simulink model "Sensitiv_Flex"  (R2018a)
settings: Solver=ode113  StartTime=0.0  StopTime=20  FixedStep=0.0001  RelTol=1e-5  EnableMultiTasking=on
InitFcn:
  | init
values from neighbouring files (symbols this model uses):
  d2r = pi/180    (= 0.0174532925199)    [init.m]    (also in LQR_Design.m)
  Kr = Kq; Kr(3)=-Kq(3)    [init.m]
  r2d = 1/d2r    (= 57.2957795131)    [init.m]    (also in LQR_Design.m)
  Wf = 18    [init.m]
undefined symbols (not defined in the file or in its folder): Aa, Av, Ba, Bv, Ca, Cv, Da, Dv, Kq, TVC

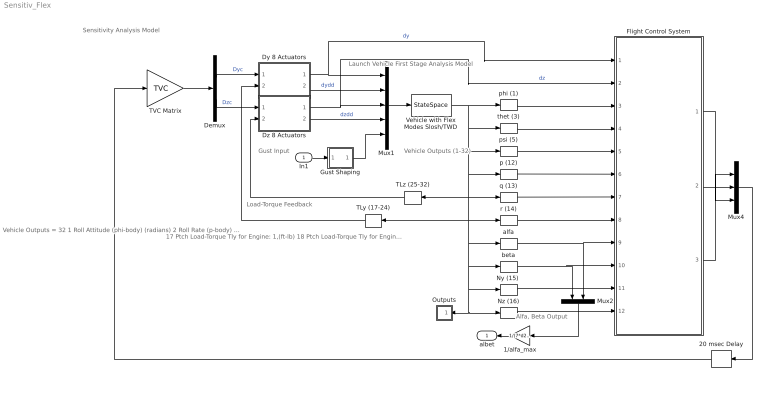
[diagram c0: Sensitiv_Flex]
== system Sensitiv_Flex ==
  note: Gust Input
  note: Launch Vehicle First Stage Analysis Model
  note: Load-Torque Feedback
  note: 17 Ptch Load-Torque Tly for Engine: 1,(ft-lb) 18 Ptch Load-Torque Tly for Engine: 2,(ft-lb) 19 Ptch Load-Torque Tly for Engine: 3,(ft-lb) 20 Ptch Load-Torque Tly for Engine: 4,(ft-lb) 21 Ptch Load-Torque Tly for Engine: 5,(ft-lb) 22 Ptch Load-Torque Tly for Engine: 6,(ft-lb) 23 Ptch Load-Torque Tly for Engine: 7,(ft-lb) 24 Ptch Load-Torque Tly for Engine: 8,(ft-lb) 25 Yaw Load-Torque Tlz for Engine: 1,(ft-lb) 26 Yaw Load-Torque Tlz for Engine: 2,(ft-lb) 27 Yaw Load-Torque Tlz for Engine: 3,(ft-lb) 28 Yaw Load-Torque Tlz for Engine: 4,(ft-lb) 29 Yaw Load-Torque Tlz for Engine: 5,(ft-lb) 30 Yaw Load-Torque Tlz for Engine: 6,(ft-lb) 31 Yaw Load-Torque Tlz for Engine: 7,(ft-lb) 32 Yaw Load-Torque Tlz for Engine: 8,(ft-lb)
  note: Vehicle Outputs = 32 1 Roll Attitude (phi-body) (radians) 2 Roll Rate (p-body) (rad/sec) 3 Pitch Attitude (thet-bdy) (radians) 4 Pitch Rate (q-body) (rad/sec) 5 Yaw Attitude (psi-body) (radians) 6 Yaw Rate (r-body) (rad/sec) 7 Angle of attack, alfa, (radians) 8 Angle of sideslip, beta, (radian) 9 Change in Altitude, delta-h, (feet) 10 Forward Acceleration (V-dot) (ft/sec) 11 Cross Range Velocity (Vcr) (ft/sec) 12 Rate-Gyro # 1, Roll Rate (Body) (rad/sec) 13 Rate-Gyro # 2, Pitch Rate (Body) (rad/sec) 14 Rate-Gyro # 3, Yaw Rate (Body) (rad/sec) 15 Accelerom # 1, (along Y), (ft/sec^2) Translat. Accelerat. 16 Accelerom # 2, (along Z), (ft/sec^2) Translat. Accelerat.
  note: Vehicle Outputs (1-32)
  note: Sensitivity Analysis Model
  note: Alfa, Beta Output
  In1 : Inport
  1/alfa_max : Gain  Gain=1/(7*d2r)
  20 msec Delay : TransportDelay  DelayTime="[1  1  1]*0.02"  InitialOutput="[0  0  0]"  PadeOrder=2
  Demux : Demux  Outputs=[8, 8]
  Dy 8 Actuators : Subsystem
  Dz 8 Actuators : Subsystem
  Flight Control System : Subsystem
  Gust Shaping : Subsystem
  Mux1 : Mux  Inputs=[8, 8, 8, 8, 1]
  Mux2 : Mux  Inputs=2
  Mux4 : Mux  Inputs=3
  "Ny (15) " : Selector  InputPortWidth=32  IndexOptions=Index vector (dialog)  Indices=[15]  OutputSizes=1
  Nz (16) : Selector  InputPortWidth=32  IndexOptions=Index vector (dialog)  Indices=[16]  OutputSizes=1
  Outputs : Subsystem
  TLy (17-24) : Selector  InputPortWidth=32  IndexOptions=Index vector (dialog)  Indices=[17:24]  OutputSizes=1
  TLz (25-32) : Selector  InputPortWidth=32  IndexOptions=Index vector (dialog)  Indices=[25:32]  OutputSizes=1
  TVC Matrix : Gain  Gain=TVC  Multiplication=Matrix(K*u)
  Vehicle with Flex Modes Slosh/TWD : StateSpace  A=Av  B=Bv  C=Cv  D=Dv  InitialCondition=0
  alfa : Selector  InputPortWidth=32  IndexOptions=Index vector (dialog)  Indices=[7]  OutputSizes=1
  beta : Selector  InputPortWidth=32  IndexOptions=Index vector (dialog)  Indices=[8]  OutputSizes=1
  p (12) : Selector  InputPortWidth=32  IndexOptions=Index vector (dialog)  Indices=[12]  OutputSizes=1
  phi (1) : Selector  InputPortWidth=32  IndexOptions=Index vector (dialog)  Indices=[1]  OutputSizes=1
  psi (5) : Selector  InputPortWidth=32  IndexOptions=Index vector (dialog)  Indices=[5]  OutputSizes=1
  q (13) : Selector  InputPortWidth=32  IndexOptions=Index vector (dialog)  Indices=[13]  OutputSizes=1
  r (14) : Selector  InputPortWidth=32  IndexOptions=Index vector (dialog)  Indices=[14]  OutputSizes=1
  thet (3) : Selector  InputPortWidth=32  IndexOptions=Index vector (dialog)  Indices=[3]  OutputSizes=1
  albet : Outport
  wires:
  Mux1/1 -> Vehicle with Flex Modes Slosh/TWD/1
  Dy 8 Actuators/2(dydd) -> Mux1/2  "dydd"
  Dz 8 Actuators/2(dzdd) -> Mux1/4  "dzdd"
  Demux/1 -> Dy 8 Actuators/1(dyc)  "Dyc"
  Dy 8 Actuators/1(dy) -> Flight Control System/1(dy), Mux1/1  "dy"
  Dz 8 Actuators/1(dz) -> Flight Control System/2(dz), Mux1/3  "dz"
  Demux/2 -> Dz 8 Actuators/1(dzc)  "Dzc"
  TLy (17-24)/1 -> Dy 8 Actuators/2(TLy)
  TLz (25-32)/1 -> Dz 8 Actuators/2(TLz)
  Vehicle with Flex Modes Slosh/TWD/1 -> TLz (25-32)/1, "Ny (15) "/1, Outputs/1(in), Nz (16)/1, beta/1, alfa/1, TLy (17-24)/1, r (14)/1, q (13)/1, p (12)/1, psi (5)/1, thet (3)/1, phi (1)/1
  r (14)/1 -> Flight Control System/8(r)
  q (13)/1 -> Flight Control System/7(q)
  p (12)/1 -> Flight Control System/6(p)
  Mux4/1 -> 20 msec Delay/1
  alfa/1 -> Flight Control System/9(alfa), Mux2/2
  beta/1 -> Flight Control System/10(beta), Mux2/1
  "Ny (15) "/1 -> Flight Control System/11(NY)
  Nz (16)/1 -> Flight Control System/12(NZ)
  Flight Control System/2(DQ_tvc) -> Mux4/2
  Flight Control System/1(DP_tvc) -> Mux4/1
  Flight Control System/3(DR_tvc) -> Mux4/3
  phi (1)/1 -> Flight Control System/3(phi)
  thet (3)/1 -> Flight Control System/4(thet)
  psi (5)/1 -> Flight Control System/5(psi)
  TVC Matrix/1 -> Demux/1
  In1/1 -> Gust Shaping/1(i)
  Mux2/1 -> 1/alfa_max/1
  20 msec Delay/1 -> TVC Matrix/1
  Gust Shaping/1(o) -> Mux1/5
  1/alfa_max/1 -> albet/1

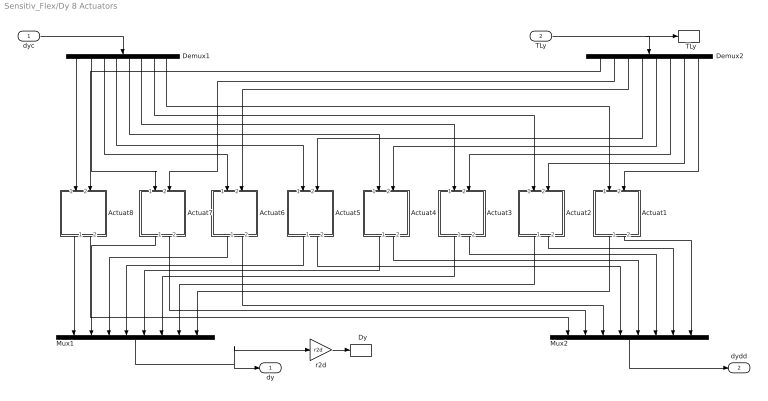
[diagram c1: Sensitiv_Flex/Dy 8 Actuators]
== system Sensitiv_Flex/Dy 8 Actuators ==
  dyc : Inport
  TLy : Inport  Port=2
  "  Dy" : ToWorkspace  VariableName=DY  SampleTime=-1
  "  TLy" : ToWorkspace  VariableName=TLy  SampleTime=-1
  Actuat1 : Subsystem
  Actuat2 : Subsystem
  Actuat3 : Subsystem
  Actuat4 : Subsystem
  Actuat5 : Subsystem
  Actuat6 : Subsystem
  Actuat7 : Subsystem
  Actuat8 : Subsystem
  Demux1 : Demux  Outputs=8
  Demux2 : Demux  Outputs=8
  Mux1 : Mux  Inputs=8
  Mux2 : Mux  Inputs=8
  r2d : Gain  Gain=r2d
  dy : Outport
  dydd : Outport  Port=2
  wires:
  TLy/1 -> "  TLy"/1, Demux2/1
  Mux2/1 -> dydd/1
  Actuat5/1(dout) -> Mux1/4
  Demux1/5 -> Actuat4/1(delin)
  Actuat3/2(ddot) -> Mux2/6
  Actuat8/1(dout) -> Mux1/1
  Demux1/4 -> Actuat5/1(delin)
  Actuat1/1(dout) -> Mux1/8
  Actuat4/2(ddot) -> Mux2/5
  Actuat4/1(dout) -> Mux1/5
  Demux2/4 -> Actuat5/2(TL)
  Demux2/6 -> Actuat3/2(TL)
  Demux2/7 -> Actuat2/2(TL)
  Actuat6/2(ddot) -> Mux2/3
  Demux2/2 -> Actuat7/2(TL)
  Actuat5/2(ddot) -> Mux2/4
  Demux1/3 -> Actuat6/1(delin)
  Actuat2/2(ddot) -> Mux2/7
  Actuat8/2(ddot) -> Mux2/1
  dyc/1 -> Demux1/1
  Mux1/1 -> r2d/1, dy/1
  Actuat1/2(ddot) -> Mux2/8
  Actuat7/2(ddot) -> Mux2/2
  Demux1/2 -> Actuat7/1(delin)
  Demux1/7 -> Actuat2/1(delin)
  Demux1/8 -> Actuat1/1(delin)
  Actuat7/1(dout) -> Mux1/2
  Demux2/5 -> Actuat4/2(TL)
  Demux1/1 -> Actuat8/1(delin)
  Demux2/1 -> Actuat8/2(TL)
  Actuat2/1(dout) -> Mux1/7
  Demux2/8 -> Actuat1/2(TL)
  Demux2/3 -> Actuat6/2(TL)
  Actuat3/1(dout) -> Mux1/6
  Actuat6/1(dout) -> Mux1/3
  Demux1/6 -> Actuat3/1(delin)
  r2d/1 -> "  Dy"/1

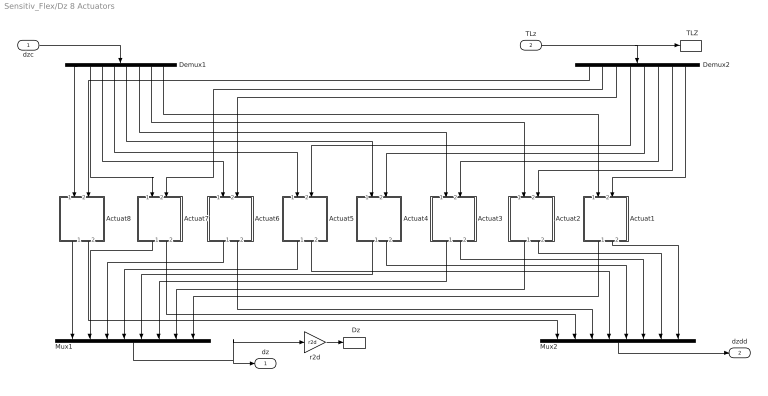
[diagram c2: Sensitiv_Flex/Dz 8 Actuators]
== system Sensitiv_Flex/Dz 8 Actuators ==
  dzc : Inport
  TLz : Inport  Port=2
  "  Dz" : ToWorkspace  VariableName=DZ  SampleTime=-1
  "  TLZ" : ToWorkspace  VariableName=TLz  SampleTime=-1
  Actuat1 : Subsystem
  Actuat2 : Subsystem
  Actuat3 : Subsystem
  Actuat4 : Subsystem
  Actuat5 : Subsystem
  Actuat6 : Subsystem
  Actuat7 : Subsystem
  Actuat8 : Subsystem
  Demux1 : Demux  Outputs=8
  Demux2 : Demux  Outputs=8
  Mux1 : Mux  Inputs=8
  Mux2 : Mux  Inputs=8
  r2d : Gain  Gain=r2d
  dz : Outport
  dzdd : Outport  Port=2
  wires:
  TLz/1 -> "  TLZ"/1, Demux2/1
  Mux2/1 -> dzdd/1
  Actuat5/1(dout) -> Mux1/4
  Demux1/5 -> Actuat4/1(delin)
  Actuat3/2(ddot) -> Mux2/6
  Actuat8/1(dout) -> Mux1/1
  Demux1/4 -> Actuat5/1(delin)
  Actuat1/1(dout) -> Mux1/8
  Actuat4/2(ddot) -> Mux2/5
  Actuat4/1(dout) -> Mux1/5
  Demux2/4 -> Actuat5/2(TL)
  Demux2/6 -> Actuat3/2(TL)
  Demux2/7 -> Actuat2/2(TL)
  Actuat6/2(ddot) -> Mux2/3
  Demux2/2 -> Actuat7/2(TL)
  Actuat5/2(ddot) -> Mux2/4
  Demux1/3 -> Actuat6/1(delin)
  Actuat2/2(ddot) -> Mux2/7
  Actuat8/2(ddot) -> Mux2/1
  dzc/1 -> Demux1/1
  Mux1/1 -> r2d/1, dz/1
  Actuat1/2(ddot) -> Mux2/8
  Actuat7/2(ddot) -> Mux2/2
  Demux1/2 -> Actuat7/1(delin)
  Demux1/7 -> Actuat2/1(delin)
  Demux1/8 -> Actuat1/1(delin)
  Actuat7/1(dout) -> Mux1/2
  Demux2/5 -> Actuat4/2(TL)
  Demux1/1 -> Actuat8/1(delin)
  Demux2/1 -> Actuat8/2(TL)
  Actuat2/1(dout) -> Mux1/7
  Demux2/8 -> Actuat1/2(TL)
  Demux2/3 -> Actuat6/2(TL)
  Actuat3/1(dout) -> Mux1/6
  Actuat6/1(dout) -> Mux1/3
  Demux1/6 -> Actuat3/1(delin)
  r2d/1 -> "  Dz"/1

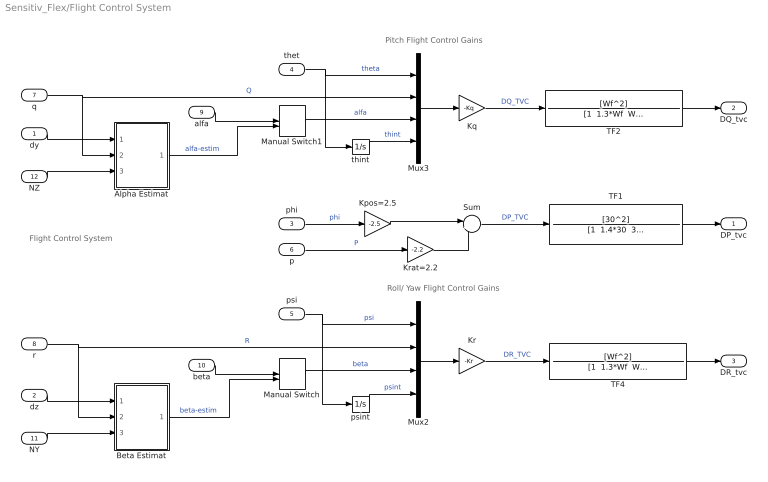
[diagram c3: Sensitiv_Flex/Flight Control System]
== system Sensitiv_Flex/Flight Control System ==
  note: Pitch Flight Control Gains
  note: Roll/ Yaw Flight Control Gains
  note: Flight Control System
  dy : Inport
  dz : Inport  Port=2
  phi : Inport  Port=3
  thet : Inport  Port=4
  psi : Inport  Port=5
  p : Inport  Port=6
  q : Inport  Port=7
  r : Inport  Port=8
  alfa : Inport  Port=9
  beta : Inport  Port=10
  NY : Inport  Port=11
  NZ : Inport  Port=12
  Alpha Estimat : Subsystem
  Beta Estimat : Subsystem
  Kpos=2.5 : Gain  Gain=-2.5  Multiplication=Matrix(K*u)
  Kq : Gain  Gain=-Kq  Multiplication=Matrix(K*u)
  Kr : Gain  Gain=-Kr  Multiplication=Matrix(K*u)
  Krat=2.2 : Gain  Gain=-2.2  Multiplication=Matrix(K*u)
  Manual Switch : ManualSwitch  CurrentSetting=0
  Manual Switch1 : ManualSwitch  CurrentSetting=0
  Mux2 : Mux
  Mux3 : Mux
  Sum : Sum  Inputs=|++
  TF1 : TransferFcn  Numerator=[30^2]  Denominator="[1  1.4*30  30^2]"
  TF2 : TransferFcn  Numerator=[Wf^2]  Denominator="[1  1.3*Wf  Wf^2]"
  TF4 : TransferFcn  Numerator=[Wf^2]  Denominator="[1  1.3*Wf  Wf^2]"
  psint : Integrator
  thint : Integrator
  DP_tvc : Outport
  DQ_tvc : Outport  Port=2
  DR_tvc : Outport  Port=3
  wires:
  Alpha Estimat/1(alfest) -> Manual Switch1/2  "alfa-estim"
  alfa/1 -> Manual Switch1/1
  Manual Switch1/1 -> Mux3/3  "alfa"
  beta/1 -> Manual Switch/1
  Manual Switch/1 -> Mux2/3  "beta"
  psi/1 -> psint/1, Mux2/1  "psi"
  psint/1 -> Mux2/4  "psint"
  q/1 -> Alpha Estimat/2(q), Mux3/2  "Q"
  r/1 -> Beta Estimat/2(r), Mux2/2  "R"
  thint/1 -> Mux3/4  "thint"
  Kr/1 -> TF4/1  "DR_TVC"
  thet/1 -> thint/1, Mux3/1  "theta"
  Kq/1 -> TF2/1  "DQ_TVC"
  TF4/1 -> DR_tvc/1
  TF2/1 -> DQ_tvc/1
  NZ/1 -> Alpha Estimat/3(Zdd)
  NY/1 -> Beta Estimat/3(Ydd)
  Beta Estimat/1(betest) -> Manual Switch/2  "beta-estim"
  dy/1 -> Alpha Estimat/1(dy)
  dz/1 -> Beta Estimat/1(dz)
  Mux3/1 -> Kq/1
  Kpos=2.5/1 -> Sum/1
  Sum/1 -> TF1/1  "DP_TVC"
  Krat=2.2/1 -> Sum/2
  p/1 -> Krat=2.2/1  "P"
  phi/1 -> Kpos=2.5/1  "phi"
  Mux2/1 -> Kr/1
  TF1/1 -> DP_tvc/1

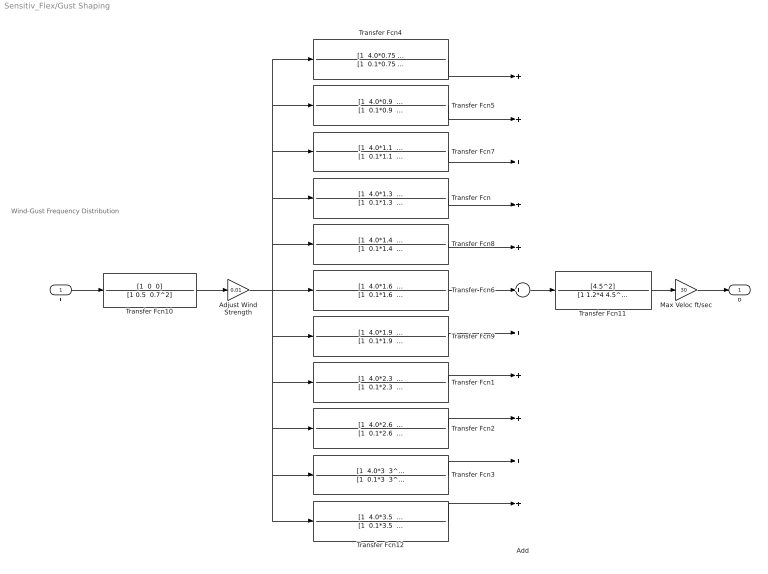
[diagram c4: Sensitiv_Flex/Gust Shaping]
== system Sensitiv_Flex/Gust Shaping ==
  note: Wind-Gust Frequency Distribution
  i : Inport
  Add : Sum  Inputs=+++++++++++
  Adjust Wind Strength : Gain  Gain=0.01
  Max Veloc ft/sec : Gain  Gain=30
  Transfer Fcn : TransferFcn  Numerator="[1  4.0*1.3  1.3^2]"  Denominator="[1  0.1*1.3  1.3^2]"
  Transfer Fcn1 : TransferFcn  Numerator="[1  4.0*2.3  2.3^2]"  Denominator="[1  0.1*2.3  2.3^2]"
  Transfer Fcn10 : TransferFcn  Numerator="[1  0  0]"  Denominator="[1 0.5  0.7^2]"
  Transfer Fcn11 : TransferFcn  Numerator=[4.5^2]  Denominator=[1 1.2*4 4.5^2]
  Transfer Fcn12 : TransferFcn  Numerator="[1  4.0*3.5  3.5^2]"  Denominator="[1  0.1*3.5  3.5^2]"
  Transfer Fcn2 : TransferFcn  Numerator="[1  4.0*2.6  2.6^2]"  Denominator="[1  0.1*2.6  2.6^2]"
  Transfer Fcn3 : TransferFcn  Numerator="[1  4.0*3  3^2]"  Denominator="[1  0.1*3  3^2]"
  Transfer Fcn4 : TransferFcn  Numerator="[1  4.0*0.75  0.75^2]"  Denominator="[1  0.1*0.75  0.75^2]"
  Transfer Fcn5 : TransferFcn  Numerator="[1  4.0*0.9  0.9^2]"  Denominator="[1  0.1*0.9  0.9^2]"
  Transfer Fcn6 : TransferFcn  Numerator="[1  4.0*1.6  1.6^2]"  Denominator="[1  0.1*1.6  1.6^2]"
  Transfer Fcn7 : TransferFcn  Numerator="[1  4.0*1.1  1.1^2]"  Denominator="[1  0.1*1.1  1.1^2]"
  Transfer Fcn8 : TransferFcn  Numerator="[1  4.0*1.4  1.4^2]"  Denominator="[1  0.1*1.4  1.4^2]"
  Transfer Fcn9 : TransferFcn  Numerator="[1  4.0*1.9  1.9^2]"  Denominator="[1  0.1*1.9  1.9^2]"
  o : Outport
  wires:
  Transfer Fcn9/1 -> Add/7
  Transfer Fcn10/1 -> Adjust Wind Strength/1
  Add/1 -> Transfer Fcn11/1
  Transfer Fcn2/1 -> Add/9
  Transfer Fcn8/1 -> Add/5
  Transfer Fcn5/1 -> Add/2
  i/1 -> Transfer Fcn10/1
  Transfer Fcn4/1 -> Add/1
  Transfer Fcn7/1 -> Add/3
  Transfer Fcn6/1 -> Add/6
  Transfer Fcn/1 -> Add/4
  Transfer Fcn3/1 -> Add/10
  Transfer Fcn1/1 -> Add/8
  Transfer Fcn12/1 -> Add/11
  Transfer Fcn11/1 -> Max Veloc ft/sec/1
  Adjust Wind Strength/1 -> Transfer Fcn6/1, Transfer Fcn5/1, Transfer Fcn4/1, Transfer Fcn7/1, Transfer Fcn/1, Transfer Fcn8/1, Transfer Fcn1/1, Transfer Fcn2/1, Transfer Fcn12/1, Transfer Fcn3/1, Transfer Fcn9/1
  Max Veloc ft/sec/1 -> o/1

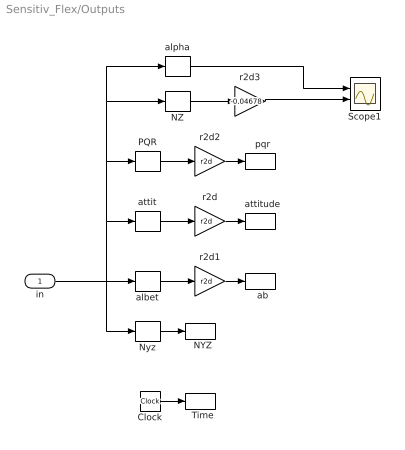
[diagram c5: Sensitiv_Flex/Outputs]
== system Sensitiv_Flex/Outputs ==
  in : Inport
  "  NYZ" : ToWorkspace  VariableName=Nyz  SampleTime=-1
  "  Time" : ToWorkspace  VariableName=tim  SampleTime=-1
  "  ab" : ToWorkspace  VariableName=albet  SampleTime=-1
  "  attitude" : ToWorkspace  VariableName=atti  SampleTime=-1
  "  pqr" : ToWorkspace  VariableName=pqr  SampleTime=-1
  Clock : Clock
  NZ : Selector  InputPortWidth=32  IndexOptions=Index vector (dialog)  Indices=[16]  OutputSizes=1
  Nyz : Selector  InputPortWidth=32  IndexOptions=Index vector (dialog)  Indices=[15,16]  OutputSizes=1
  PQR : Selector  InputPortWidth=32  IndexOptions=Index vector (dialog)  Indices=[12, 13, 14]  OutputSizes=1
  Scope1 : Scope  NumInputPorts=2
  albet : Selector  InputPortWidth=32  IndexOptions=Index vector (dialog)  Indices=[7,8]  OutputSizes=1
  alpha : Selector  InputPortWidth=32  IndexOptions=Index vector (dialog)  Indices=[7]  OutputSizes=1
  attit : Selector  InputPortWidth=32  IndexOptions=Index vector (dialog)  Indices="[1  3   5]"  OutputSizes=1
  r2d : Gain  Gain=r2d
  r2d1 : Gain  Gain=r2d
  r2d2 : Gain  Gain=r2d
  r2d3 : Gain  Gain=-0.04678
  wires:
  alpha/1 -> Scope1/1
  r2d3/1 -> Scope1/2
  NZ/1 -> r2d3/1
  r2d2/1 -> "  pqr"/1
  PQR/1 -> r2d2/1
  Clock/1 -> "  Time"/1
  r2d1/1 -> "  ab"/1
  r2d/1 -> "  attitude"/1
  attit/1 -> r2d/1
  in/1 -> albet/1, Nyz/1, attit/1, PQR/1, alpha/1, NZ/1
  Nyz/1 -> "  NYZ"/1
  albet/1 -> r2d1/1

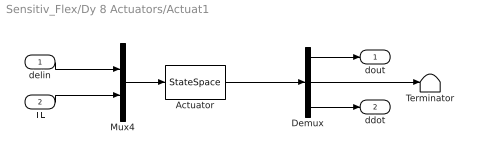
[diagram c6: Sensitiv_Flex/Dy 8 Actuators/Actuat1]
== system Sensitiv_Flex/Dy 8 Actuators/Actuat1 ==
  delin : Inport
  TL : Inport  Port=2
  Actuator : StateSpace  A=Aa  B=Ba  C=Ca  D=Da  InitialCondition=0
  Demux : Demux  Outputs=3
  Mux4 : Mux  Inputs=2
  Terminator : Terminator
  dout : Outport
  ddot : Outport  Port=2
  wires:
  Demux/3 -> ddot/1
  TL/1 -> Mux4/2
  Mux4/1 -> Actuator/1
  Actuator/1 -> Demux/1
  delin/1 -> Mux4/1
  Demux/1 -> dout/1
  Demux/2 -> Terminator/1

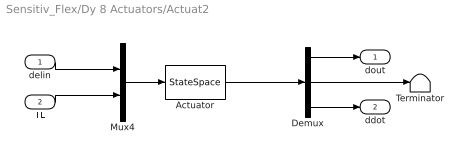
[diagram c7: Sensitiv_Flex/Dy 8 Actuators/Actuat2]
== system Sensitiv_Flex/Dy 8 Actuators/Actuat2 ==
  delin : Inport
  TL : Inport  Port=2
  Actuator : StateSpace  A=Aa  B=Ba  C=Ca  D=Da  InitialCondition=0
  Demux : Demux  Outputs=3
  Mux4 : Mux  Inputs=2
  Terminator : Terminator
  dout : Outport
  ddot : Outport  Port=2
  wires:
  Demux/3 -> ddot/1
  TL/1 -> Mux4/2
  Mux4/1 -> Actuator/1
  Actuator/1 -> Demux/1
  delin/1 -> Mux4/1
  Demux/1 -> dout/1
  Demux/2 -> Terminator/1

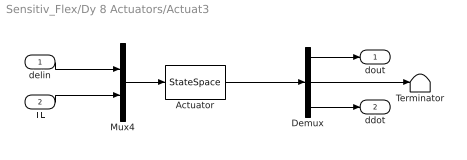
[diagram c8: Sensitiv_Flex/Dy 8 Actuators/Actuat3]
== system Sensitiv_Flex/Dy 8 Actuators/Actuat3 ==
  delin : Inport
  TL : Inport  Port=2
  Actuator : StateSpace  A=Aa  B=Ba  C=Ca  D=Da  InitialCondition=0
  Demux : Demux  Outputs=3
  Mux4 : Mux  Inputs=2
  Terminator : Terminator
  dout : Outport
  ddot : Outport  Port=2
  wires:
  Demux/3 -> ddot/1
  TL/1 -> Mux4/2
  Mux4/1 -> Actuator/1
  Actuator/1 -> Demux/1
  delin/1 -> Mux4/1
  Demux/1 -> dout/1
  Demux/2 -> Terminator/1

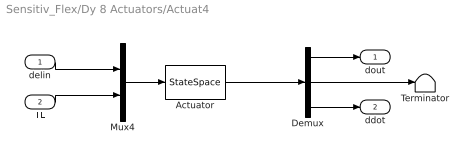
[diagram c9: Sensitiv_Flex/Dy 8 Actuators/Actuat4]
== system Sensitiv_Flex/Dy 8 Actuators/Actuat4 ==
  delin : Inport
  TL : Inport  Port=2
  Actuator : StateSpace  A=Aa  B=Ba  C=Ca  D=Da  InitialCondition=0
  Demux : Demux  Outputs=3
  Mux4 : Mux  Inputs=2
  Terminator : Terminator
  dout : Outport
  ddot : Outport  Port=2
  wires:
  Demux/3 -> ddot/1
  TL/1 -> Mux4/2
  Mux4/1 -> Actuator/1
  Actuator/1 -> Demux/1
  delin/1 -> Mux4/1
  Demux/1 -> dout/1
  Demux/2 -> Terminator/1

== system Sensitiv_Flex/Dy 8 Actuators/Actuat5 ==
  delin : Inport
  TL : Inport  Port=2
  Actuator : StateSpace  A=Aa  B=Ba  C=Ca  D=Da  InitialCondition=0
  Demux : Demux  Outputs=3
  Mux4 : Mux  Inputs=2
  Terminator : Terminator
  dout : Outport
  ddot : Outport  Port=2
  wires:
  Demux/3 -> ddot/1
  TL/1 -> Mux4/2
  Mux4/1 -> Actuator/1
  Actuator/1 -> Demux/1
  delin/1 -> Mux4/1
  Demux/1 -> dout/1
  Demux/2 -> Terminator/1

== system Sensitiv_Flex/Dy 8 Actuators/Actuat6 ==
  delin : Inport
  TL : Inport  Port=2
  Actuator : StateSpace  A=Aa  B=Ba  C=Ca  D=Da  InitialCondition=0
  Demux : Demux  Outputs=3
  Mux4 : Mux  Inputs=2
  Terminator : Terminator
  dout : Outport
  ddot : Outport  Port=2
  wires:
  Demux/3 -> ddot/1
  TL/1 -> Mux4/2
  Mux4/1 -> Actuator/1
  Actuator/1 -> Demux/1
  delin/1 -> Mux4/1
  Demux/1 -> dout/1
  Demux/2 -> Terminator/1

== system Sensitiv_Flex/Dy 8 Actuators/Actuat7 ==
  delin : Inport
  TL : Inport  Port=2
  Actuator : StateSpace  A=Aa  B=Ba  C=Ca  D=Da  InitialCondition=0
  Demux : Demux  Outputs=3
  Mux4 : Mux  Inputs=2
  Terminator : Terminator
  dout : Outport
  ddot : Outport  Port=2
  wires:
  Demux/3 -> ddot/1
  TL/1 -> Mux4/2
  Mux4/1 -> Actuator/1
  Actuator/1 -> Demux/1
  delin/1 -> Mux4/1
  Demux/1 -> dout/1
  Demux/2 -> Terminator/1

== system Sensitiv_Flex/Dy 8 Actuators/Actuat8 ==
  delin : Inport
  TL : Inport  Port=2
  Actuator : StateSpace  A=Aa  B=Ba  C=Ca  D=Da  InitialCondition=0
  Demux : Demux  Outputs=3
  Mux4 : Mux  Inputs=2
  Terminator : Terminator
  dout : Outport
  ddot : Outport  Port=2
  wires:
  Demux/3 -> ddot/1
  TL/1 -> Mux4/2
  Mux4/1 -> Actuator/1
  Actuator/1 -> Demux/1
  delin/1 -> Mux4/1
  Demux/1 -> dout/1
  Demux/2 -> Terminator/1

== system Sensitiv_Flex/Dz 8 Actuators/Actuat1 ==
  delin : Inport
  TL : Inport  Port=2
  Actuator : StateSpace  A=Aa  B=Ba  C=Ca  D=Da  InitialCondition=0
  Demux : Demux  Outputs=3
  Mux4 : Mux  Inputs=2
  Terminator : Terminator
  dout : Outport
  ddot : Outport  Port=2
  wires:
  Demux/3 -> ddot/1
  TL/1 -> Mux4/2
  Mux4/1 -> Actuator/1
  Actuator/1 -> Demux/1
  delin/1 -> Mux4/1
  Demux/1 -> dout/1
  Demux/2 -> Terminator/1

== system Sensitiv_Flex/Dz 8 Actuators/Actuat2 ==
  delin : Inport
  TL : Inport  Port=2
  Actuator : StateSpace  A=Aa  B=Ba  C=Ca  D=Da  InitialCondition=0
  Demux : Demux  Outputs=3
  Mux4 : Mux  Inputs=2
  Terminator : Terminator
  dout : Outport
  ddot : Outport  Port=2
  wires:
  Demux/3 -> ddot/1
  TL/1 -> Mux4/2
  Mux4/1 -> Actuator/1
  Actuator/1 -> Demux/1
  delin/1 -> Mux4/1
  Demux/1 -> dout/1
  Demux/2 -> Terminator/1

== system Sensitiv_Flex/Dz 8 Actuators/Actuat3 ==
  delin : Inport
  TL : Inport  Port=2
  Actuator : StateSpace  A=Aa  B=Ba  C=Ca  D=Da  InitialCondition=0
  Demux : Demux  Outputs=3
  Mux4 : Mux  Inputs=2
  Terminator : Terminator
  dout : Outport
  ddot : Outport  Port=2
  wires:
  Demux/3 -> ddot/1
  TL/1 -> Mux4/2
  Mux4/1 -> Actuator/1
  Actuator/1 -> Demux/1
  delin/1 -> Mux4/1
  Demux/1 -> dout/1
  Demux/2 -> Terminator/1

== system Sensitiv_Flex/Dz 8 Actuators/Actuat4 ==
  delin : Inport
  TL : Inport  Port=2
  Actuator : StateSpace  A=Aa  B=Ba  C=Ca  D=Da  InitialCondition=0
  Demux : Demux  Outputs=3
  Mux4 : Mux  Inputs=2
  Terminator : Terminator
  dout : Outport
  ddot : Outport  Port=2
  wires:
  Demux/3 -> ddot/1
  TL/1 -> Mux4/2
  Mux4/1 -> Actuator/1
  Actuator/1 -> Demux/1
  delin/1 -> Mux4/1
  Demux/1 -> dout/1
  Demux/2 -> Terminator/1

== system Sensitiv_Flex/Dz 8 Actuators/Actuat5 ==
  delin : Inport
  TL : Inport  Port=2
  Actuator : StateSpace  A=Aa  B=Ba  C=Ca  D=Da  InitialCondition=0
  Demux : Demux  Outputs=3
  Mux4 : Mux  Inputs=2
  Terminator : Terminator
  dout : Outport
  ddot : Outport  Port=2
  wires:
  Demux/3 -> ddot/1
  TL/1 -> Mux4/2
  Mux4/1 -> Actuator/1
  Actuator/1 -> Demux/1
  delin/1 -> Mux4/1
  Demux/1 -> dout/1
  Demux/2 -> Terminator/1

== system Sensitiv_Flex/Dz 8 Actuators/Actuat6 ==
  delin : Inport
  TL : Inport  Port=2
  Actuator : StateSpace  A=Aa  B=Ba  C=Ca  D=Da  InitialCondition=0
  Demux : Demux  Outputs=3
  Mux4 : Mux  Inputs=2
  Terminator : Terminator
  dout : Outport
  ddot : Outport  Port=2
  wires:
  Demux/3 -> ddot/1
  TL/1 -> Mux4/2
  Mux4/1 -> Actuator/1
  Actuator/1 -> Demux/1
  delin/1 -> Mux4/1
  Demux/1 -> dout/1
  Demux/2 -> Terminator/1

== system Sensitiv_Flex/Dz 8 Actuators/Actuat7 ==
  delin : Inport
  TL : Inport  Port=2
  Actuator : StateSpace  A=Aa  B=Ba  C=Ca  D=Da  InitialCondition=0
  Demux : Demux  Outputs=3
  Mux4 : Mux  Inputs=2
  Terminator : Terminator
  dout : Outport
  ddot : Outport  Port=2
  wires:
  Demux/3 -> ddot/1
  TL/1 -> Mux4/2
  Mux4/1 -> Actuator/1
  Actuator/1 -> Demux/1
  delin/1 -> Mux4/1
  Demux/1 -> dout/1
  Demux/2 -> Terminator/1

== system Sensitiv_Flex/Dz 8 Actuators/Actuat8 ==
  delin : Inport
  TL : Inport  Port=2
  Actuator : StateSpace  A=Aa  B=Ba  C=Ca  D=Da  InitialCondition=0
  Demux : Demux  Outputs=3
  Mux4 : Mux  Inputs=2
  Terminator : Terminator
  dout : Outport
  ddot : Outport  Port=2
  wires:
  Demux/3 -> ddot/1
  TL/1 -> Mux4/2
  Mux4/1 -> Actuator/1
  Actuator/1 -> Demux/1
  delin/1 -> Mux4/1
  Demux/1 -> dout/1
  Demux/2 -> Terminator/1

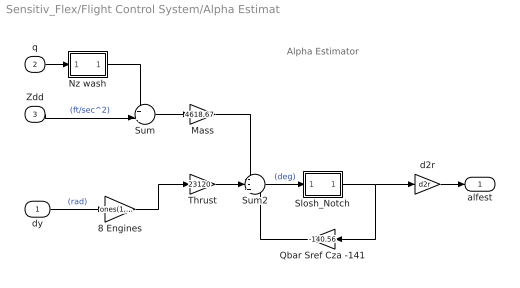
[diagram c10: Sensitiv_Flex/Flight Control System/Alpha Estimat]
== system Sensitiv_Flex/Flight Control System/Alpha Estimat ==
  note: Alpha Estimator
  dy : Inport
  q : Inport  Port=2
  Zdd : Inport  Port=3
  8 Engines : Gain  Gain=ones(1,8)  Multiplication=Matrix(K*u) (u vector)
  Mass : Gain  Gain=4618.67
  Nz wash : Subsystem
  Qbar Sref Cza -141 : Gain  Gain=-140.56
  Slosh_Notch : Subsystem
  Sum : Sum  Inputs=++|
  Sum2 : Sum  Inputs=--+
  Thrust : Gain  Gain=23120
  d2r : Gain  Gain=d2r
  alfest : Outport
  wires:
  8 Engines/1 -> Thrust/1
  Mass/1 -> Sum2/1
  Slosh_Notch/1(ou) -> Qbar Sref Cza -141/1, d2r/1
  Nz wash/1(ou) -> Sum/1
  Sum2/1 -> Slosh_Notch/1(in)  "(deg)"
  Qbar Sref Cza -141/1 -> Sum2/3
  Zdd/1 -> Sum/2  "(ft/sec^2)"
  d2r/1 -> alfest/1
  q/1 -> Nz wash/1(in)
  Sum/1 -> Mass/1
  dy/1 -> 8 Engines/1  "(rad)"
  Thrust/1 -> Sum2/2

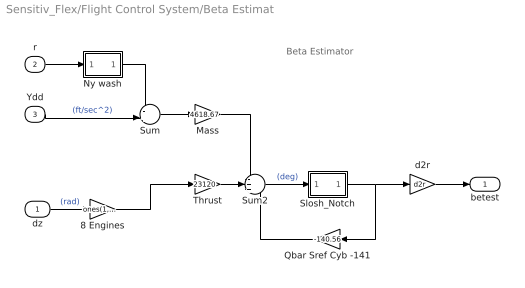
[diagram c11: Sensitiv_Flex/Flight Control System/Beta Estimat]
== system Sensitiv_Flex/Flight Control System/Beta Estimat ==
  note: Beta Estimator
  dz : Inport
  r : Inport  Port=2
  Ydd : Inport  Port=3
  8 Engines : Gain  Gain=ones(1,8)  Multiplication=Matrix(K*u) (u vector)
  Mass : Gain  Gain=4618.67
  Ny wash : Subsystem
  Qbar Sref Cyb -141 : Gain  Gain=-140.56
  Slosh_Notch : Subsystem
  Sum : Sum  Inputs=-+|
  Sum2 : Sum  Inputs=-++
  Thrust : Gain  Gain=23120
  d2r : Gain  Gain=d2r
  betest : Outport
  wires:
  8 Engines/1 -> Thrust/1
  dz/1 -> 8 Engines/1  "(rad)"
  Slosh_Notch/1(ou) -> d2r/1, Qbar Sref Cyb -141/1
  Ny wash/1(ou) -> Sum/1
  Sum2/1 -> Slosh_Notch/1(in)  "(deg)"
  Qbar Sref Cyb -141/1 -> Sum2/3
  Ydd/1 -> Sum/2  "(ft/sec^2)"
  Mass/1 -> Sum2/1
  d2r/1 -> betest/1
  Thrust/1 -> Sum2/2
  r/1 -> Ny wash/1(in)
  Sum/1 -> Mass/1

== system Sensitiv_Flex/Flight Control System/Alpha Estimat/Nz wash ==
  in : Inport
  3 : Gain  Gain=19
  Transfer Fcn : TransferFcn  Numerator="[1  0]"  Denominator="[0.015  1]"
  ou : Outport
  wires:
  3/1 -> ou/1
  Transfer Fcn/1 -> 3/1
  in/1 -> Transfer Fcn/1

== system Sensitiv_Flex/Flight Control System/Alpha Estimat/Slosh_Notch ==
  in : Inport
  0.1 : Gain  Gain=0.0015
  Int1 : Integrator
  Transfer Fcn1 : TransferFcn  Numerator="[1 0.015*4  3.72^2]"  Denominator="[1  0.3*4  3.72^2]"
  ou : Outport
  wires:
  Transfer Fcn1/1 -> Int1/1
  0.1/1 -> Transfer Fcn1/1
  Int1/1 -> ou/1
  in/1 -> 0.1/1

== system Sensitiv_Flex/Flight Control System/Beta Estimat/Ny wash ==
  in : Inport
  3 : Gain  Gain=19
  Transfer Fcn1 : TransferFcn  Numerator="[1  0]"  Denominator="[0.015  1]"
  ou : Outport
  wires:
  3/1 -> ou/1
  Transfer Fcn1/1 -> 3/1
  in/1 -> Transfer Fcn1/1

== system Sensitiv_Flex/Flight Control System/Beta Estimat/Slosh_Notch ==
  in : Inport
  0.1 : Gain  Gain=0.0015
  Int1 : Integrator
  Transfer Fcn2 : TransferFcn  Numerator="[1 0.015*4  3.72^2]"  Denominator="[1  0.3*4  3.72^2]"
  ou : Outport
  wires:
  Transfer Fcn2/1 -> Int1/1
  0.1/1 -> Transfer Fcn2/1
  Int1/1 -> ou/1
  in/1 -> 0.1/1
